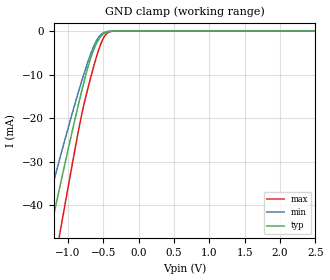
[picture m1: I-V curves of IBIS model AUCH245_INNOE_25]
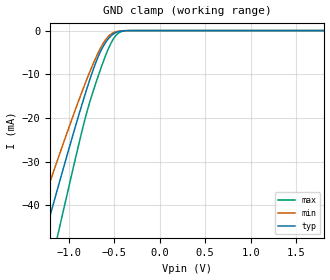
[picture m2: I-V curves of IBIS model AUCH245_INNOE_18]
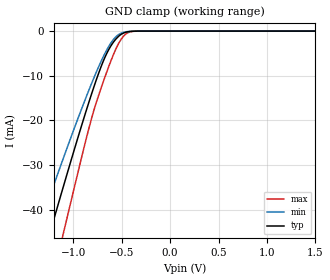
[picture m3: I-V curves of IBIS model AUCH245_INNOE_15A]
| TEXAS INSTRUMENTS INCORPORATED
| Standard Linear and Logic Group
| IBIS Model of SN74AUCH245
| Octal Bus Transceiver with 3-State Outputs
| This file contains package information for the following:
|  QFN 20-pin (RGY) package as [Component] SN74AUCH245_RGY
| This device can be powered at the following Vccs:
|  2.5 volt Vcc
|  1.8 volt Vcc
|  1.5 volt Vcc
|  1.2 volt Vcc
|  0.8 volt Vcc
| This file provides unique models under the [Model Selector] for each Vcc.
| For operation at a specific Vcc, select the appropriate model after each
| [Model Selector] keyword.
[IBIS Ver]   3.2
[Comment char]  |_char
[File Name]   sn74auch245.ibs
[File Rev]   1.1 | x_die
[Date]   March 22, 2007
[Source]   Data created from TI-SPICE simulations at TI-SLL.
[Notes]   The following is an IBIS list for the SN74AUCH245.
   Please contact sllibis@ti.com with questions and
   comments concerning SLL IBIS models.
   - FILE REV HISTORY
   - 1.1 IBIS file released on 03/29/07
   - Power clamp data deleted as there is no power-clamp diode.
   - End point warning due to AC and DC mismatch.
   - Non-monotonic data in ground-clamp due to bus-hold
   - The waveform abnormalities for the AUCH245_IO Power Clamp,
   Pullup, and Pulldown are caused by the circuitry that helps
   reduce overshoot and undershoot in transmission lines (EMI).
   These waveforms are normal for this particular design.
[Disclaimer] Property of Texas Instruments Incorporated.  Unauthorized
   reproduction and/or distribution is strictly prohibited.
   This product is protected under copyright law.
   Created  2007, (C) Copyright  2007, Texas Instruments
   Incorporated, All Rights Reserved
   UNLESS THERE IS A SIGNED, WRITTEN AGREEMENT TO THE
   CONTRARY, TEXAS INSTRUMENTS (TI) IS PROVIDING THE IBIS
   MODELS  AND WITHOUT ANY WARRANTY, EXPRESSED OR
   IMPLIED.  TI assumes no liability for:
   1) the accuracy of the IBIS models provided to your
   company;
   2) the proper functioning of these IBIS Models in your
   design or for any resulting applications; or
   3) infringement of patents, copyrights or intellectual
   property rights resulting from your use of these IBIS
   models.
   TI provides IBIS Models as a service to our customers.
   You and your company shall not distribute, sell or give
   these models to anyone else without prior written
   permission from TI.
   TI reserves the right to make changes to our products or
   to discontinue any semiconductor product or service
   without notice, and advises our customers to obtain the
   latest version of relevant information to verify, before
   placing orders, that the information being relied on is
   current.
   Please be aware that your receipt and use of the IBIS
   information provided shall serve as acceptance of these
   terms and conditions.  If you do not accept these terms,
   you should return or destroy the IBIS models and any
   other accompanying information immediately.
| Component SN74AUCH245_RGY 20-PIN QFN
[Component]   SN74AUCH245_RGY
[Manufacturer]   Texas Instruments, Inc.
[Package]
|   typ   min   max
R_pkg   5.000e-02   4.600e-02   5.500e-02
L_pkg   1.119e-09   1.025e-09   1.227e-09
C_pkg   3.520e-13   3.440e-13   3.630e-13
[Pin]   signal_name   model_name   R_pin   L_pin   C_pin
1   DIR   AUCH245_INDIR   5.200e-02   1.167e-09   3.600e-13
2   A1   AUCH245_IO   4.700e-02   1.049e-09   3.440e-13
3   A2   AUCH245_IO   4.700e-02   1.055e-09   3.450e-13
4   A3   AUCH245_IO   5.000e-02   1.119e-09   3.500e-13
5   A4   AUCH245_IO   5.500e-02   1.227e-09   3.600e-13
6   A5   AUCH245_IO   5.200e-02   1.167e-09   3.550e-13
7   A6   AUCH245_IO   4.900e-02   1.087e-09   3.480e-13
8   A7   AUCH245_IO   4.700e-02   1.054e-09   3.460e-13
9   A8   AUCH245_IO   4.900e-02   1.091e-09   3.490e-13
10   GND   GND   5.300e-02   1.184e-09   3.620e-13
11   B8   AUCH245_IO   5.300e-02   1.181e-09   3.600e-13
12   B7   AUCH245_IO   5.000e-02   1.108e-09   3.490e-13
13   B6   AUCH245_IO   4.800e-02   1.075e-09   3.470e-13
14   B5   AUCH245_IO   5.000e-02   1.107e-09   3.490e-13
15   B4   AUCH245_IO   5.400e-02   1.200e-09   3.620e-13
16   B3   AUCH245_IO   5.100e-02   1.141e-09   3.570e-13
17   B2   AUCH245_IO   4.700e-02   1.043e-09   3.440e-13
18   B1   AUCH245_IO   4.600e-02   1.025e-09   3.440e-13
19   NOE   AUCH245_INNOE   4.900e-02   1.090e-09   3.490e-13
20   VCC   POWER   5.400e-02   1.204e-09   3.630e-13
| Model AUCH245_INNOE
[Model Selector]   AUCH245_INNOE
AUCH245_INNOE_25   2.5 volt Vcc
AUCH245_INNOE_18   1.8 volt Vcc
AUCH245_INNOE_15A   1.5 volt Vcc
AUCH245_INNOE_12   1.2 volt Vcc
AUCH245_INNOE_08   0.8 volt Vcc
| Model AUCH245_INDIR
[Model Selector]   AUCH245_INDIR
AUCH245_INDIR_25   2.5 volt Vcc
AUCH245_INDIR_18   1.8 volt Vcc
AUCH245_INDIR_15A   1.5 volt Vcc
AUCH245_INDIR_12   1.2 volt Vcc
AUCH245_INDIR_08   0.8 volt Vcc
| Model AUCH245_IO
[Model Selector]   AUCH245_IO
AUCH245_IO_25   2.5 volt Vcc
AUCH245_IO_18   1.8 volt Vcc
AUCH245_IO_15A   1.5 volt Vcc
AUCH245_IO_12   1.2 volt Vcc
AUCH245_IO_08   0.8 volt Vcc
| Models and submodels in the file (15): AUCH245_INNOE_25 (Input), AUCH245_INNOE_18 (Input), AUCH245_INNOE_15A (Input), AUCH245_INNOE_12 (Input), AUCH245_INNOE_08 (Input), AUCH245_INDIR_25 (Input), AUCH245_INDIR_18 (Input), AUCH245_INDIR_15A (Input), AUCH245_INDIR_12 (Input), AUCH245_INDIR_08 (Input), AUCH245_IO_25 (3-state), AUCH245_IO_18 (3-state), AUCH245_IO_15A (3-state), AUCH245_IO_12 (3-state), AUCH245_IO_08 (3-state)
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[Model]   AUCH245_INNOE_25
Model_type  Input
Vinl=0.7
Vinh=1.7
| variable   typ   min   max
C_comp   2.47pF   1.97pF   2.92pF
[Temperature Range]   40   100   -40
| Ambient temperature   25   85   -40
[Voltage range]   2.5   2.3   2.7
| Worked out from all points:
|   GND clamp passes 1 mA (typ) near -0.52 V on its own axis
[GND Clamp]
| AUCH245_INNOE_25
|   Voltage   I(typ)   I(min)   I(max)
-3.6V     -229.3mA   -192.6mA   -273mA
-1.38V    -55.83mA   -45.62mA   -70.82mA
-1.28V    -48.21mA   -39.37mA   -61.64mA
-1.235V   -44.81mA   -36.59mA   -57.52mA
-1.11V    -35.45mA   -28.97mA   -46.07mA
-830mV    -15.39mA   -12.79mA   -21.13mA
-710mV    -7.848mA   -6.681mA   -12.62mA
-600mV    -2.951mA   -2.314mA   -6.078mA
-490mV    -542.1uA   -342.5uA   -1.378mA
-430mV    -133.4uA   -89.21uA   -324.3uA
-340mV    -10.37uA   -9.319uA   -15.22uA
2.5V      453pA      1.243nA    77.67pA
[Model]   AUCH245_INNOE_18
Model_type  Input
Vinl=0.5775
Vinh=1.2675
| variable   typ   min   max
C_comp   2.54pF   2.06pF   2.97pF
[Temperature Range]   40   100   -40
| Ambient temperature   25   85   -40
[Voltage range]   1.8   1.65   1.95
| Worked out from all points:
|   GND clamp passes 1 mA (typ) near -0.52 V on its own axis
[GND Clamp]
| AUCH245_INNOE_18
|   Voltage   I(typ)   I(min)   I(max)
-3.6V     -229.3mA   -192.6mA   -273mA
-1.425V   -59.27mA   -48.46mA   -74.95mA
-1.375V   -55.44mA   -45.31mA   -70.36mA
-1.28V    -48.21mA   -39.37mA   -61.64mA
-1.235V   -44.81mA   -36.59mA   -57.52mA
-1.12V    -36.19mA   -29.57mA   -46.99mA
-1.085V   -33.6mA    -27.46mA   -43.79mA
-815mV    -14.38mA   -11.99mA   -19.92mA
-695mV    -7.027mA   -5.991mA   -11.68mA
-550mV    -1.561mA   -1.085mA   -3.576mA
-450mV    -220uA     -142.1uA   -557.1uA
1.8V      305pA      941.6pA    47.06pA
[Model]   AUCH245_INNOE_15A
Model_type  Input
Vinl=0.49
Vinh=1.04
| variable   typ   min   max
C_comp   2.57pF   2.11pF   3.03pF
[Temperature Range]   40   100   -40
| Ambient temperature   25   85   -40
[Voltage range]   1.5   1.4   1.6
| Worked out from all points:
|   GND clamp passes 1 mA (typ) near -0.52 V on its own axis
[GND Clamp]
| AUCH245_INNOE_15A
|   Voltage   I(typ)   I(min)   I(max)
-3.6V     -229.3mA   -192.6mA   -273mA
-1.365V   -54.68mA   -44.68mA   -69.45mA
-1.23V    -44.43mA   -36.28mA   -57.06mA
-1.11V    -35.45mA   -28.97mA   -46.07mA
-1.065V   -32.12mA   -26.27mA   -41.97mA
-815mV    -14.38mA   -11.99mA   -19.92mA
-700mV    -7.296mA   -6.219mA   -11.99mA
-585mV    -2.484mA   -1.884mA   -5.281mA
-515mV    -880.3uA   -569.4uA   -2.161mA
-460mV    -279.4uA   -178.2uA   -714.3uA
-315mV    -4.754uA   -4.767uA   -5.622uA
1.5V      253.5pA    827.7pA    37.14pA
